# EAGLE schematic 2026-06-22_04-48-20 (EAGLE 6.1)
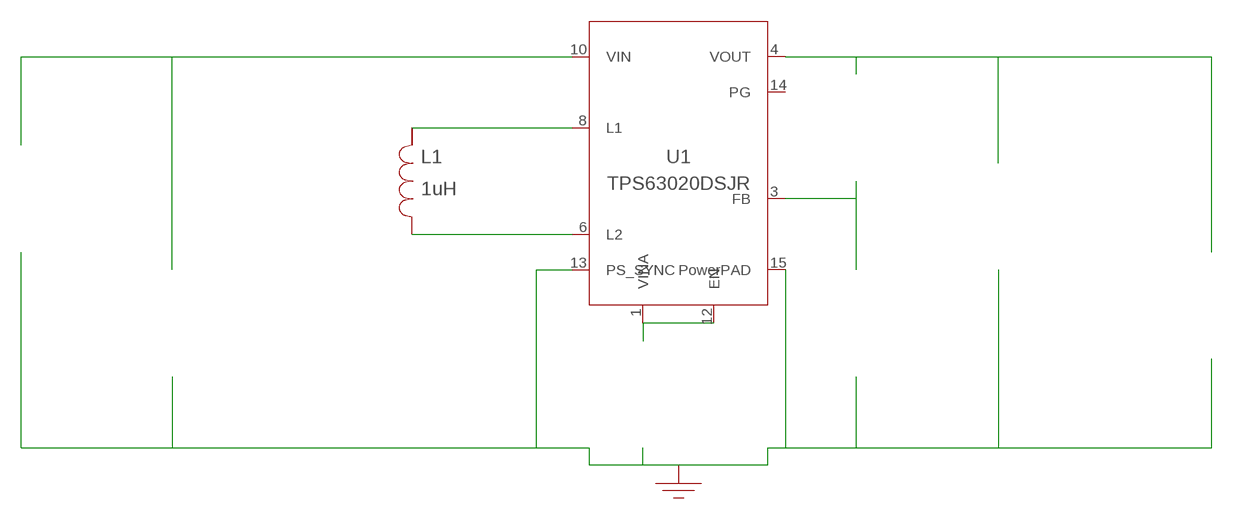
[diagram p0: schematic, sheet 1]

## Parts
CIN  22uF  C1608X5R1A226M080ACC1608X5R1A226M080AC  [0603]  (not placed on a sheet)
COUT  47uF  MSASJ21GBB5476MTNA01MSASJ21GBB5476MTNA01  [0805]  (not placed on a sheet)
CVINA  100nF  EMK107B7104KA-TEMK107B7104KA-T  [0603]  (not placed on a sheet)
GND  WB_GND  WB_GNDWB_GND  [WB_GND]
IOUT  WB_CURRENT_LOAD  WB_CURRENT_LOADWB_CURRENT_LOAD  [WB_CURRENT_LOAD]  (not placed on a sheet)
L1  1uH  DFE201610E-1R0M=P2DFE201610E-1R0M=P2  [GEN_Ind]
RFBB  137k  CRCW0402137KFKEDCRCW0402137KFKED  [0402]  (not placed on a sheet)
RFBT  768k  CRCW0402768KFKEDCRCW0402768KFKED  [0402]  (not placed on a sheet)
U1  TPS63020DSJR  TPS63020DSJRTPS63020DSJR  [R-PVSON-N14]
VIN  WB_BATTERY  WB_BATTERYWB_BATTERY  [WB_BATTERY]  (not placed on a sheet)
Unconnected: CIN.1 CIN.2 COUT.1 COUT.2 CVINA.1 CVINA.2 GND.1 IOUT.1(+) IOUT.2(-) L1.1 L1.2 RFBB.1 RFBB.2 RFBT.1 RFBT.2 U1.1(VINA) U1.2(GND) U1.3(FB) U1.4(VOUT) U1.5(VOUT) U1.6(L2) U1.7(L2) U1.8(L1) U1.9(L1) U1.10(VIN) U1.11(VIN) U1.12(EN) U1.13(PS_SYNC) U1.14(PG) U1.15(PowerPAD) VIN.1(+) VIN.2(-)

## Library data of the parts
CIN = AcceleratedDesigns_Lib:C1608X5R1A226M080AC; Manufacturer_Part_Number: C1608X5R1A226M080AC; Vendor: TDK
COUT = AcceleratedDesigns_Lib:MSASJ21GBB5476MTNA01; Manufacturer_Part_Number: MSASJ21GBB5476MTNA01; Vendor: Taiyo Yuden
CVINA = AcceleratedDesigns_Lib:EMK107B7104KA-T; Manufacturer_Part_Number: EMK107B7104KA-T; Vendor: Taiyo Yuden
GND = AcceleratedDesigns_Lib:WB_GND; Manufacturer_Part_Number: WB_GND
IOUT = AcceleratedDesigns_Lib:WB_CURRENT_LOAD; Manufacturer_Part_Number: WB_CURRENT_LOAD
L1 = AcceleratedDesigns_Lib:DFE201610E-1R0M=P2; Manufacturer_Part_Number: GENERIC_INDUCTOR; Vendor: Unknown
RFBB = AcceleratedDesigns_Lib:CRCW0402137KFKED; Manufacturer_Part_Number: CRCW0402137KFKED; Vendor: Vishay-Dale
RFBT = AcceleratedDesigns_Lib:CRCW0402768KFKED; Manufacturer_Part_Number: CRCW0402768KFKED; Vendor: Vishay-Dale
U1 = AcceleratedDesigns_Lib:TPS63020DSJR; Manufacturer_Part_Number: TPS63020DSJR; Vendor: Texas Instruments
VIN = AcceleratedDesigns_Lib:WB_BATTERY; Manufacturer_Part_Number: WB_BATTERY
